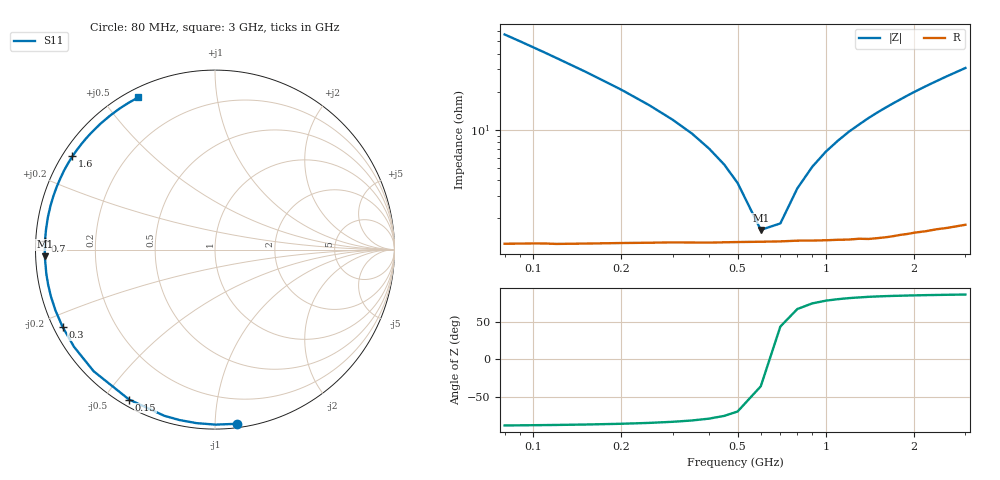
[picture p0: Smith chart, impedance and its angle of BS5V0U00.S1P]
! SIEMENS Small Signal Semiconductors
! BB640
! Si Tuning Diode in SOD323
! VR = 5 V
! S-Parameters:  July  1993
# GHz  S  MA  R  50
!  f  S11
! GHz  MAG  ANG
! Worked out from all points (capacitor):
!   33 points, 80 MHz to 3 GHz, reference 50 ohm
!   read as one part to ground: C = 34.6 pF near 80 MHz
!   lowest |Z| = 1.62 ohm at 600 MHz (marker M1)
!   series resonance near 643.1 MHz, so ESL is about 1.8 nH
!   S11 on the Smith chart (normalised r, x): 80 MHz: 0.03, -1.13; 150 MHz: 0.03, -0.58; 300 MHz: 0.03, -0.24; 700 MHz: 0.03, +0.03; 1.6 GHz: 0.03, +0.30; 3 GHz: 0.04, +0.61
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0.08  0.9781 -82.9
0.09  0.9751 -89.8
0.1  0.9723 -96.1
0.11  0.9699 -101.8
0.12  0.968 -107.0
0.15  0.9628 -119.8
0.2  0.9573 -134.9
0.25  0.9542 -145.4
0.3  0.9522 -153.1
0.35  0.9513 -159.1
0.4  0.9507 -164.1
0.45  0.95 -168.2
0.5  0.9495 -171.8
0.6  0.949 -177.8
0.7  0.9487 177.1
0.8  0.9482 172.7
0.9  0.9484 168.7
1  0.9485 165.0
1.2  0.9488 158.3
1.4  0.9494 152.3
1.6  0.9492 146.8
1.8  0.9484 141.7
2  0.9481 136.8
2.2  0.9483 132.3
2.4  0.9482 128.1
2.6  0.9488 124.1
2.8  0.9491 120.4
3  0.9496 116.8
